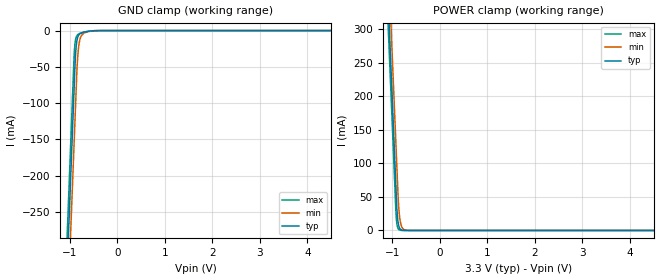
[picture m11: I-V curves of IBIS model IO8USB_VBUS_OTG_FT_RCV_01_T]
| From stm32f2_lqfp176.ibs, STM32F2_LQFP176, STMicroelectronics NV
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| *** New cell (Generated with 5.14beta1 (Sep 20 2010 13:23:23))
[Model]   IO8USB_VBUS_OTG_FT_RCV_01_T
Model_type Input
Polarity   Non-Inverting
Enable   Active-Low
| CAP_THRESHOLD on pad IOV33 is "CMOS" :
| Rising=10.0% of vdd5   Falling=90.0% of vdd5
| C_comp min and max val. don't necessarily correlate with the min and max pvt
| but are the smallest and greatest pad capacitance found.
| var   typ   min   max
C_comp   2.69340pF  2.58200pF  2.86325pF
Vinl = 800.0mV | Dummy value overriden by next lines
Vinh = 2.00V | Dummy value overriden by next lines
[Model Spec]
| TIME_THRESHOLD on pin ZIV33 is "CORE" :
| Rising=40.0% of vddio   Falling=60.0% of vddio
Vinl 1.25450V 1.03850V 1.36250V
Vinh 1.66150V 1.36950V 1.82450V
| variable   typ   min   max
[Temperature Range] 25.0 125.0 -40.0
| variable   typ   min   max
[Voltage Range] 3.3V 2.7V 3.6V
| variable   typ   min   max
[POWER Clamp Reference] 3.3V 2.7V 3.6V
| variable   typ   min   max
[GND Clamp Reference] 0V 0V 0V
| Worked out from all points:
|   GND clamp passes 1 mA (typ) near -0.61 V on its own axis
|   POWER clamp passes 1 mA (typ) near -0.81 V on its own axis
[POWER Clamp]
-3.3V     4.11A      4.173A     4.072A
-1.09V    352.5mA    415.9mA    314.5mA
-1.05V    284.5mA    347.9mA    246.5mA
-1.01V    216.5mA    279.9mA    178.5mA
-920mV    63.51mA    126.9mA    25.85mA
-900mV    31.51mA    92.9mA     9.552mA
-890mV    21.35mA    75.9mA     5.807mA
-870mV    9.804mA    44.01mA    2.146mA
-840mV    3.05mA     18.36mA    482.1uA
-780mV    295.2uA    3.193mA    24.34uA
-660mV    2.764uA    96.47uA    62.42nA
6.6V      0A         0A         0A
[GND Clamp]
-3.3V     -4.149A    -4.224A    -4.103A
-1.06V    -341.2mA   -416.1mA   -295.1mA
-940mV    -137.2mA   -212.1mA   -91.08mA
-900mV    -69.19mA   -144.1mA   -27.04mA
-880mV    -37.32mA   -110.1mA   -13.88mA
-870mV    -27.09mA   -93.14mA   -10.66mA
-840mV    -11.71mA   -45.57mA   -6.266mA
-820mV    -7.587mA   -27.56mA   -5.077mA
-790mV    -4.752mA   -13.78mA   -4.031mA
-700mV    -2.155mA   -3.174mA   -2.051mA
-350mV    -10.35uA   -54.26uA   -1.982uA
6.6V      13.96nA    1.746uA    94.44pA
